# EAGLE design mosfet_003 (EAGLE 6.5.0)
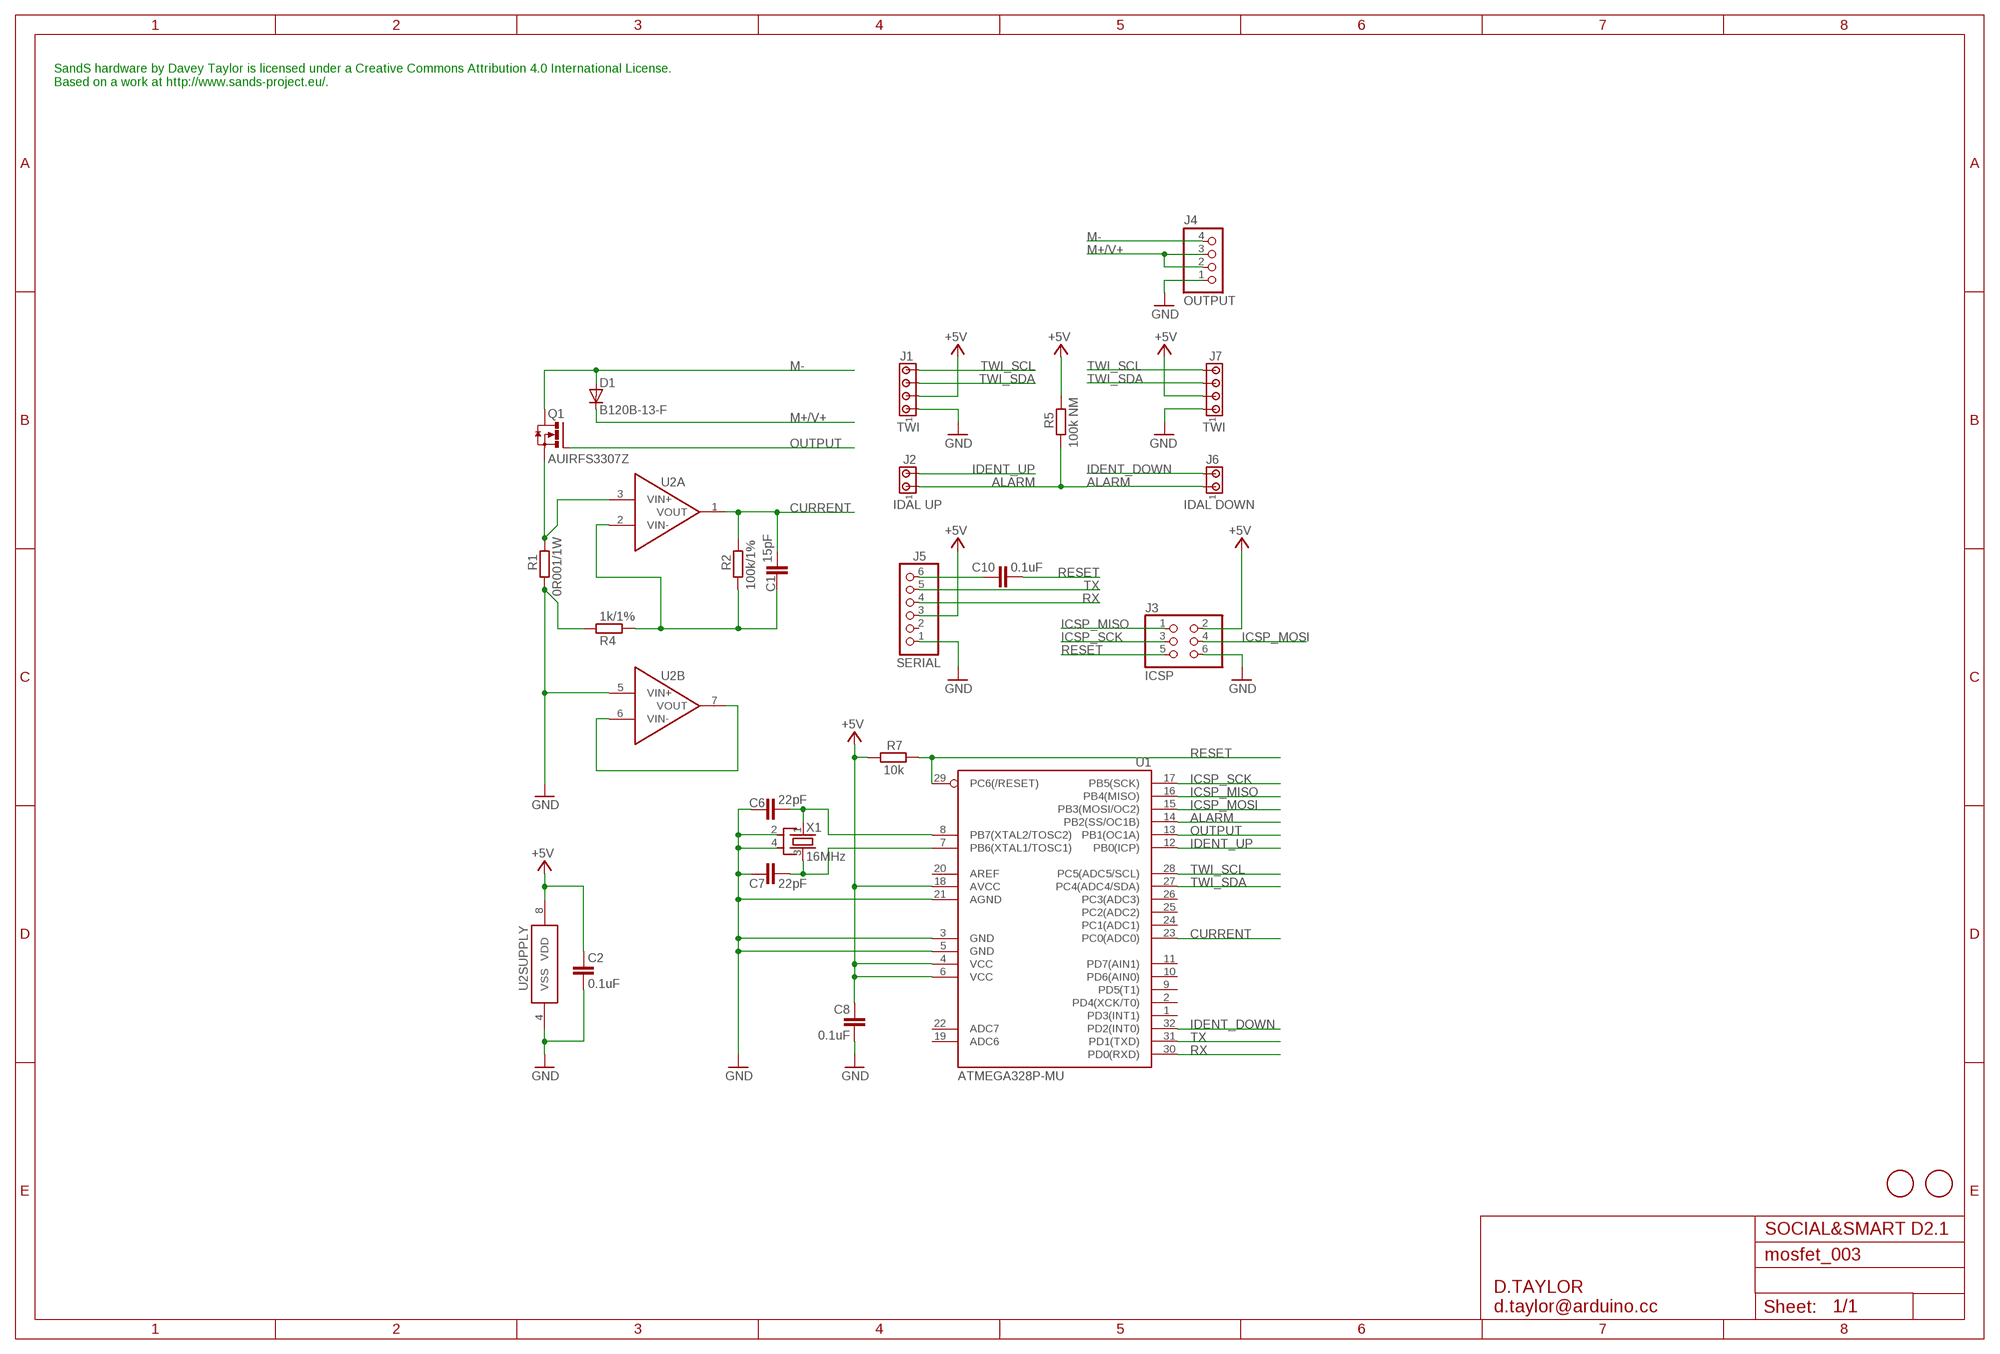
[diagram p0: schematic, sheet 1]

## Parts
C1  15pF  C-EUC0603  [C0603]
C2  0.1uF  C-EUC0603  [C0603]
C6  22pF  C-EUC0603  [C0603]
C7  22pF  C-EUC0603  [C0603]
C8  0.1uF  C-EUC0603  [C0603]
C10  0.1uF  C-EUC0603  [C0603]
D1  B120B-13-F  DIODE-SMB  [SMB]
J1  TWI  MTA04-100  [10X04MTA]
J2  IDAL UP  MTA02-100  [10X02MTA]
J3  ICSP  PINHD-2X3  [2X03]
J4  OUTPUT  MKDS_1,5/4-5,08  [MKDS1,5/4-5,08]
J5  SERIAL  PINHD-1X6  [1X06]
J6  IDAL DOWN  MTA02-100  [10X02MTA]
J7  TWI  MTA04-100  [10X04MTA]
Q1  AUIRFS3307Z  [D2PACK]
R1  0R001/1W  R-EU_R2512  [R2512]
R2  100k/1%  R-EU_R0603  [R0603]
R4  1k/1%  R-EU_R0603  [R0603]
R5  100k NM  R-EU_R0603  [R0603]
R7  10k  R-EU_R0603  [R0603]
U1  ATMEGA328P-MU  [MLF32-M1-A]
U2  LTC6081  [MSOP08]
U$5  FIDUCIALMOUNT  [FIDUCIA-MOUNT]
U$6  FIDUCIALMOUNT  [FIDUCIA-MOUNT]
X1  16MHz  CRYSTAL-KX7  [XTAL-3.2-2.5]

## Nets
+5V: C2.1 C8.1 J1.2 J3.2 J5.3 J7.2 R5.2 R7.1 U1.4(VCC) U1.6(VCC) U1.18(AVCC) U2.8(SUPPLY:VDD)
ALARM: J2.1 J6.1 R5.1 U1.14(PB2(SS/OC1B))
CURRENT: C1.2 R2.2 U1.23(PC0(ADC0)) U2.1(A:VOUT)
GND: C2.2 C6.1 C7.1 C8.2 J1.1 J3.6 J4.1 J5.1 J7.1 R1.1 R4.2 U1.3(GND) U1.5(GND) U1.21(AGND) U2.4(SUPPLY:VSS) U2.5(B:VIN+) X1.2(SH1) X1.4(SH2)
ICSP_MISO: J3.1 U1.16(PB4(MISO))
ICSP_MOSI: J3.4 U1.15(PB3(MOSI/OC2))
ICSP_SCK: J3.3 U1.17(PB5(SCK))
IDENT_DOWN: J6.2 U1.32(PD2(INT0))
IDENT_UP: J2.2 U1.12(PB0(ICP))
M+/V+: D1.C J4.2 J4.3
M-: D1.A J4.4 Q1.2(D)
N$1: Q1.3(S) R1.2 U2.3(A:VIN+)
N$2: U2.6(B:VIN-) U2.7(B:VOUT)
N$3: C1.1 R2.1 R4.1 U2.2(A:VIN-)
N$6: C6.2 U1.8(PB7(XTAL2/TOSC2)) X1.1(X1)
N$7: C7.2 U1.7(PB6(XTAL1/TOSC1)) X1.3(X2)
N$9: C10.1 J5.6
OUTPUT: Q1.1(G) U1.13(PB1(OC1A))
RESET: C10.2 J3.5 R7.2 U1.29(PC6(/RESET))
RX: J5.4 U1.30(PD0(RXD))
TWI_SCL: J1.4 J7.4 U1.28(PC5(ADC5/SCL))
TWI_SDA: J1.3 J7.3 U1.27(PC4(ADC4/SDA))
TX: J5.5 U1.31(PD1(TXD))
Unconnected: J5.2 U1.1(PD3(INT1)) U1.2(PD4(XCK/T0)) U1.9(PD5(T1)) U1.10(PD6(AIN0)) U1.11(PD7(AIN1)) U1.19(ADC6) U1.20(AREF) U1.22(ADC7) U1.24(PC1(ADC1)) U1.25(PC2(ADC2)) U1.26(PC3(ADC3))

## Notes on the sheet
- SandS hardware by Davey Taylor is licensed under a Creative Commons Attribution 4.0 International License.
  Based on a work at http://www.sands-project.eu/.
- SOCIAL&SMART D2.1
- D.TAYLOR
  d.taylor@arduino.cc

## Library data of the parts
C1 C2 C6-C8 C10 = rcl:C-EU: CAPACITOR, European symbol
D1 = diode:DIODE-: DIODE
J1 J7 = con-amp:MTA04-100: AMP connector
J2 J6 = con-amp:MTA02-100: AMP connector
J3 = pinhead:PINHD-2X3: PIN HEADER
J4 = d_taylor:MKDS_1,5/4-5,08
J5 = pinhead:PINHD-1X6: PIN HEADER
Q1 = d_taylor:AUIRFS3307: SMPS MOSFET HEXFET® Power MOSFET Source: http://www.irf.com/product-info/datasheets/data/irf3704.pdf
R1 R2 R4 R5 R7 = rcl:R-EU_: RESISTOR, European symbol
U1 = d_taylor:ATMEGA*: MICROCONTROLLER 8 Kbytes FLASH 1 kbytes SRAM 512 bytes EEPROM USART 6-channel 10 bit ADC 2-channel 8 bit ADC Source: avr.lbr
U2 = d_taylor:LTC6081
U$5 U$6 = SmartPrj:FIDUCIALMOUNT
X1 = d_taylor:CRYSTAL-KX7

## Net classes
1 PWR: width 0.406 mm, clearance 0.254 mm

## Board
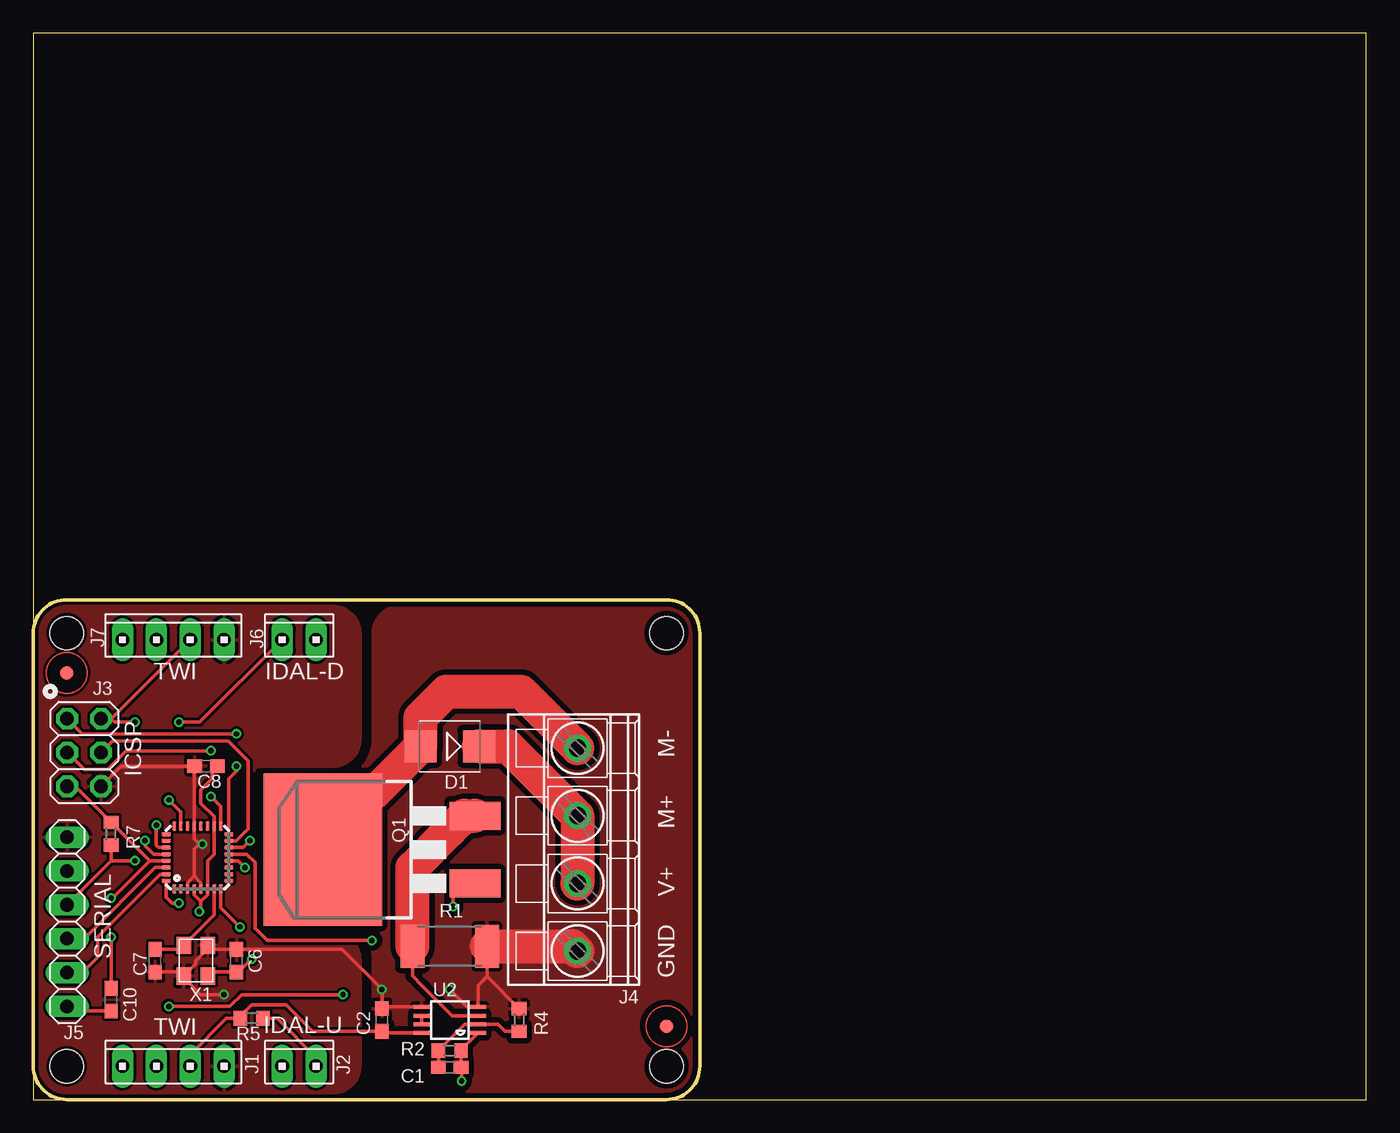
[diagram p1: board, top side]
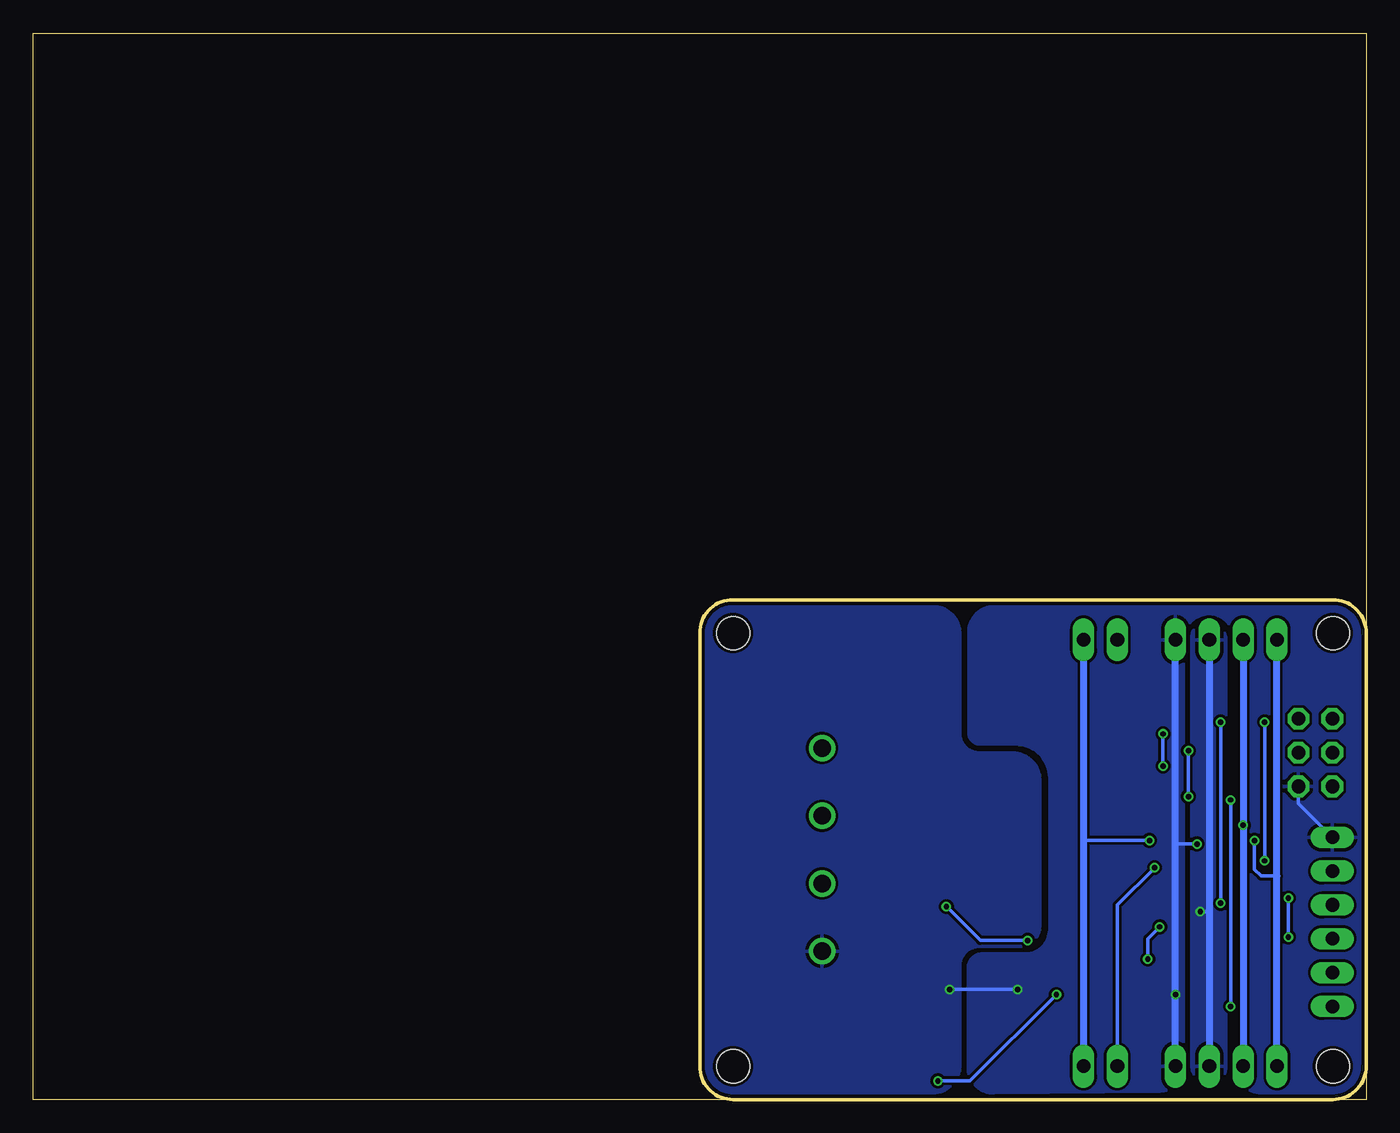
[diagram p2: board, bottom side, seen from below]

Size 100 x 80 mm. Coordinates in mm from the lower left corner, seen from the top.
Outline: 0,35 0,80 100,80 100,0 0,0 0,35
Outline: 0,35 arc-90 2.5,37.5 47.5,37.5 arc-90 50,35 50,2.5 arc-90 47.5,0 2.5,0 arc-90 0,2.5 0,35
Copper layers (1*16): Top 0.035mm / dielectric 1.5mm / Bottom 0.035mm
Design rules "smartprj-mini *": minimum track width 10mil, minimum drill 10mil, track to track 8mil, track to pad 8mil, pad to pad 0.200659375mm, via to via 8mil, smd to smd 4mil, copper to edge 10mil, drill to drill 8mil, minimum pad ring 12mil, minimum via ring 6mil, stop-mask expansion 2mil, vias tented up to drill 20mil, thermal gap 10mil
Holes 2.5 mm at 2.5,35 2.5,2.5 47.5,2.5 47.5,35

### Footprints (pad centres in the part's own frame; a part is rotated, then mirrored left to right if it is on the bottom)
C0603 = smd 1.1 x 1: 1 -0.85,0; 2 0.85,0
SMB = smd 2.4 x 2.4: A 2.2,0; C -2.2,0
10X04MTA = drill 1.016 long: 1 3.81,0; 2 1.27,0; 3 -1.27,0; 4 -3.81,0
10X02MTA = drill 1.016 long: 1 1.27,0; 2 -1.27,0
2X03 = drill 1.016 octagon: 1 -2.54,-1.27; 2 -2.54,1.27; 3 0,-1.27; 4 0,1.27; 5 2.54,-1.27; 6 2.54,1.27
MKDS1,5/4-5,08 = drill 1.3 pad 2: 1 -7.62,0; 2 -2.54,0; 3 2.54,0; 4 7.62,0
1X06 = drill 1.016 long: 1 -6.35,0; 2 -3.81,0; 3 -1.27,0; 4 1.27,0; 5 3.81,0; 6 6.35,0
D2PACK = smd 2.083 x 3.81: 1 -2.54,-8.89; 3 2.54,-8.89 | smd 11.43 x 8.89: 2 0,2.54
R2512 = smd 1.8 x 3.2: 1 -2.8,0; 2 2.8,0
R0603 = smd 1 x 1.1: 1 -0.85,0; 2 0.85,0
MLF32-M1-A = smd 0.7 x 0.3: 1 -2.35,1.75; 2 -2.35,1.25; 3 -2.35,0.75; 4 -2.35,0.25; 5 -2.35,-0.25; 6 -2.35,-0.75; 7 -2.35,-1.25; 8 -2.35,-1.75; 17 2.35,-1.75; 18 2.35,-1.25; 19 2.35,-0.75; 20 2.35,-0.25; 21 2.35,0.25; 22 2.35,0.75; 23 2.35,1.25; 24 2.35,1.75 | smd 0.3 x 0.7: 9 -1.75,-2.35; 10 -1.25,-2.35; 11 -0.75,-2.35; 12 -0.25,-2.35; 13 0.25,-2.35; 14 0.75,-2.35; 15 1.25,-2.35; 16 1.75,-2.35; 25 1.75,2.35; 26 1.25,2.35; 27 0.75,2.35; 28 0.25,2.35; 29 -0.25,2.35; 30 -0.75,2.35; 31 -1.25,2.35; 32 -1.75,2.35
MSOP08 = smd 0.3 x 1.2: 1 -0.976,-2.113; 2 -0.326,-2.113; 3 0.324,-2.113; 4 0.974,-2.113; 5 0.974,2.112; 6 0.324,2.112; 7 -0.326,2.112; 8 -0.976,2.112
FIDUCIA-MOUNT = smd 1.016 x 1.016: P$1 0,0
XTAL-3.2-2.5 = smd 1.3 x 1.1: 1 -1.15,-0.9; 2 1.15,-0.9; 3 1.15,0.9; 4 -1.15,0.9

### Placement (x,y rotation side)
C1  31.24,2.41 0 top
C2  26.16,5.97 90 top
C6  15.24,10.41 270 top
C7  9.14,10.41 90 top
C8  12.95,25.02 180 top
C10  5.84,7.49 90 top
D1  31.24,26.5 180 top
J1  10.5,2.5 0 top
J2  19.94,2.5 0 top
J3  3.81,26.04 270 top
J4  40.83,18.75 90 top
J5  2.54,13.34 270 top
J6  19.94,34.5 0 top
J7  10.5,34.5 0 top
Q1  24.25,18.75 90 top
R1  31.24,11.5 180 top
R2  31.24,3.68 0 top
R4  36.45,5.97 90 top
R5  16.38,6.1 180 top
R7  5.84,19.94 90 top
U1  12.32,18.16 90 top
U2  31.24,5.97 90 top
U$5  2.5,32 0 top
U$6  47.5,5.5 0 top
X1  12.19,10.41 90 top

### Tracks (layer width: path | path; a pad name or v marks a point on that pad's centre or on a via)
+5V  (via drill 0.41 pad 0.61)
  Top 0.254: U2.8 26.29,4.99 C2.1 20.95,5.12 18.96,7.11 16.38,7.11 15.53,6.26 R5.2 14.48,6.1 11.77,3.35 J1.2 | J7.2 5.84,28.57 | 5.84,28.57 J3.2 | J5.3 5.84,17.91 | 5.84,17.91 R7.1 | C8.1 13.46,24.64 13.42,24.6 13.42,24.09 12.57,23.24 12.57,22.23 13.57,21.23 U1.18 13.57,18.39 13.07,17.89 U1.6 13.07,15.36 12.57,14.86 | 12.57,14.86 12.07,15.36 U1.4 | 12.57,14.86 12.57,14.22 v12.45,14.1 | 5.84,17.91 v7.62,17.91 | 5.84,28.57 6.1,28.32 v7.62,28.32
  Bottom 0.254: v12.45,14.1 11.9,14.1 11.77,14.22 | v7.62,17.91 v7.62,28.32
  Bottom 0.508: J7.2 11.77,14.22 J1.2
  pour Bottom: 13.08,34.67 arc90 11.94,35.81 11.81,35.81 arc90 10.54,34.54 10.54,2.54 10.54,2.41 arc90 11.68,1.27 11.81,1.27 arc90 13.08,2.54
ALARM  (via drill 0.41 pad 0.61)
  Top 0.254: J2.1 21.21,3.14 18.29,6.1 R5.1 | U1.14 15.74,18.91 v16.26,19.43
  Bottom 0.254: v16.26,19.43 21.21,19.43
  Bottom 0.508: J6.1 21.21,19.43 J2.1
CURRENT  (via drill 0.41 pad 0.61)
  Top 0.254: U2.1 32.09,3.73 R2.2 C1.2 32.13,2.37 v32.13,1.4 | U1.23 11.07,21.57 v10.16,22.48 | v10.16,6.99 14.73,6.99 15.62,7.87 v23.24,7.87
  Bottom 0.254: v10.16,22.48 v10.16,6.99 | v23.24,7.87 29.72,1.4 v32.13,1.4
GND  (via drill 0.41 pad 0.61)
  Top 0.254: R1.1 34.04,9.23 | 34.04,9.23 R4.2 | 34.04,9.23 33.35,8.54 U2.4 32.55,6.94 v31.24,8.26 | U2.5 26.29,6.94 C2.2 v26.16,8.26 23.15,11.26 C6.1 13.39,11.26 X1.2 13.09,11.31 12.19,10.41 12.19,10.16 X1.4 | C7.1 10.99,9.56 X1.4 | U1.3 11.57,16.27 12.06,16.76 | 12.06,16.76 12.57,16.26 U1.5 | 12.06,16.76 12.07,16.77 12.07,18.8 12.45,19.18 | 12.07,24.98 C8.2 12.07,24.98 | X1.4 11.29,9.15 12.57,7.87 v14.31,7.87 | 12.07,24.98 6.57,24.98 J3.6 | 12.07,24.98 U1.21 12.07,19.55 12.45,19.18 | v12.7,19.18 12.45,19.18
  Top 2.54: R1.1 40.45,11.5 J4.1
  Bottom 0.254: v31.24,8.26 v26.16,8.26 | J3.6 5.08,22.23 J5.1 | v12.7,19.18 14.31,19.18
  Bottom 0.508: J1.1 v14.31,7.87 14.31,19.18 J7.1
  pour Top (isolate 0.406): 25.5,35 arc-90 27.5,37 47.5,37 arc-90 49.5,35 49.5,2.5 arc-90 47.5,0.5 27.5,0.5 arc-90 25.5,2.5 25.5,10.5 arc90 22.5,13.5 17.5,13.5 17.5,24 22.5,24 arc90 25.5,27
  pour Top: 0.5,35 arc-90 2.5,37 22.5,37 arc-90 24.5,35 24.5,27 arc-90 22.5,25 17,25 arc90 16.5,24.5 16.5,13 arc90 17,12.5 22.5,12.5 arc-90 24.5,10.5 24.5,2.5 arc-90 22.5,0.5 2.5,0.5 arc-90 0.5,2.5
  pour Bottom: 24.5,13 arc90 26,11.5 29,11.5 arc-90 30.5,10 30.5,2.5 arc90 32.5,0.5 47.5,0.5 arc90 49.5,2.5 49.5,35 arc90 47.5,37 32.5,37 arc90 30.5,35 30.5,27.5 arc-90 29,26 26.5,26 arc90 24.5,24
  pour Bottom: 0.5,35 arc-90 2.5,37 27.94,37 arc-90 29.82,35 29.82,27.53 arc-90 28.96,26.67 26.29,26.67 arc90 23.75,24.13 23.75,12.7 arc90 25.65,10.92 28.83,10.92 arc-90 29.84,9.91 29.84,2.29 arc-90 27.94,0.5 15.49,0.64 arc-90 13.72,2.41 13.72,34.42 arc90 11.81,36.45 arc90 9.91,34.54 9.91,2.54 arc-90 7.87,0.5 2.5,0.5 arc-90 0.5,2.5
ICSP_MISO  (via drill 0.41)
  Top 0.254: U1.16 14.67,24.07 15.24,24.64 v15.24,25.02 | v15.24,27.43 3.68,27.43 J3.1
  Bottom 0.254: v15.24,25.02 v15.24,27.43
ICSP_MOSI
  Top 0.254: J3.4 5.97,26.92 14.61,26.92 16.13,25.4 16.13,20.32 15.22,19.41 U1.15
ICSP_SCK  (via drill 0.41, 0.41 pad 0.61)
  Top 0.254: U1.17 14.07,22 v13.34,22.73 | v13.34,26.16 6.99,26.16 5.59,24.77 3.81,24.77 J3.3
  Bottom 0.254: v13.34,22.73 v13.34,26.16
IDENT_DOWN  (via drill 0.41 pad 0.61)
  Top 0.254: v10.92,28.32 12.49,28.32 J6.2 | U1.32 9.97,15.18 10.41,14.73 v10.92,14.73
  Bottom 0.254: v10.92,14.73 v10.92,28.32
IDENT_UP  (via drill 0.41 pad 0.61)
  Top 0.254: v15.88,17.4 15.37,17.91 U1.12
  Bottom 0.254: J2.2 18.67,14.61 v15.88,17.4
M+/V+
  Top 2.54: D1.C 35.62,26.5 J4.3 J4.2
M-
  Top 2.032: 21.71,19.17 Q1.2
  Top 2.54: J4.4 36.59,30.61 30.99,30.61 29.04,28.66 D1.A 21.71,19.17
N$1
  Top 0.254: R1.2 28.44,9.28 29.21,8.51 | 29.21,8.51 29.34,8.38 | U2.3 31.43,6.29 29.21,8.51
  Top 2.54: R1.2 28.44,17.39 31.24,20.19 32.34,21.29 Q1.3
N$2
  Top 0.254: U2.6 U2.7
N$3
  Top 0.254: R4.1 35.39,5.12 35.05,5.46 34.87,5.64 U2.2 32.35,5.64 R2.1 C1.1
N$6  (via drill 0.41 pad 0.61)
  Top 0.254: X1.1 13.39,9.56 C6.2 15.28,9.56 15.49,9.65 v16.38,10.54 | v15.49,12.95 14.07,14.38 U1.8
  Bottom 0.254: v16.38,10.54 16.38,12.06 v15.49,12.95
N$7
  Top 0.254: C7.2 10.99,11.26 X1.3 13.57,13.84 U1.7
N$9
  Top 0.254: J5.6 2.88,6.64 C10.1
OUTPUT  (via drill 0.41 pad 0.61)
  Top 0.254: U1.13 16.01,18.41 16.64,17.78 16.64,12.83 17.53,11.94 v25.4,11.94 | v31.5,14.48 31.5,15.24 32.47,16.21 Q1.1
  Bottom 0.254: v25.4,11.94 28.96,11.94 v31.5,14.48
RESET  (via drill 0.41 pad 0.61)
  Top 0.254: J3.5 3.14,23.5 R7.2 8.72,17.91 | U1.29 8.72,17.91 | 8.72,17.91 5.84,15.03 v5.84,15.11 | v5.84,12.19 C10.2
  Bottom 0.254: v5.84,15.11 v5.84,12.19
RX
  Top 0.254: U1.30 9.16,17.41 3.81,12.06 J5.4
TWI_SCL  (via drill 0.41 pad 0.61)
  Top 0.254: U1.28 9.02,18.41 8.38,19.05 v8.38,19.43
  Bottom 0.254: v8.38,19.43 8.38,17.27 7.87,16.76 6.69,16.76
  Bottom 0.508: J1.4 6.69,16.76 J7.4
TWI_SDA  (via drill 0.41 pad 0.61)
  Top 0.254: 9.96,18.92 U1.27 9.41,18.91 9.27,19.05 9.23,19.09 v9.23,20.57
  Bottom 0.508: J7.3 v9.23,20.57 J1.3
TX
  Top 0.254: U1.31 9.95,16.89 9.53,16.89 4.83,12.19 4.83,10.67 3.68,9.53 J5.5

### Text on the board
tPlace: TWI | IDAL-D | M- | ICSP | M+ | V+ | SERIAL | GND | TWI | IDAL-U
